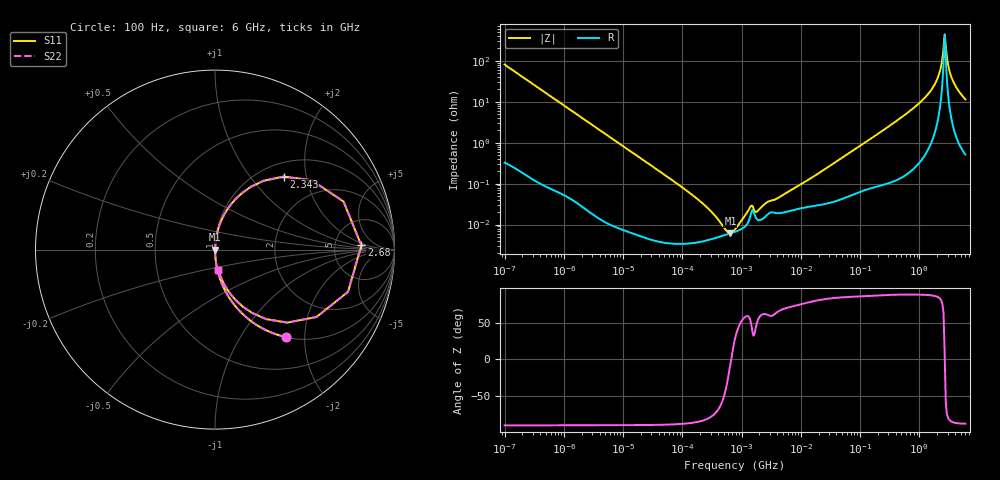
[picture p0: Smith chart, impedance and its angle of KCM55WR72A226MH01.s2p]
!Murata Part Number: KCM55WR72A226MH01
!These Parameters are Measured in Series Mode Connection
!Data Generated on Mar 13, 2026
!  o--ll--o
!Port1  Port2
!  o------o
!Operation Temp=25[degC], DC Bias Voltage=0[V]
!Freq. Start=100[Hz] Stop=6[GHz] 401[Steps]
# Hz S RI R 50
!Freq.(Hz) S11(Real) S11(Imag) S21(Real) S21(Imag) S12(Real) S12(Imag) S22(Real) S22(Imag)
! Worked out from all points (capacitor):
!   401 points, 100 Hz to 6 GHz, reference 50 ohm
!   read as one part in series: C = 19.6 uF near 109 Hz
!   lowest |Z| = 6.13 mohm at 647.6 kHz (marker M1)
!   series resonance near 665.1 kHz, so ESL is about 2.9 nH
!   S11 on the Smith chart (normalised r, x): 100 Hz: 1.01, -1.62; 2.343 GHz: 1.26, +1.49; 2.68 GHz: 9.67, +1.36; 6 GHz: 1.01, -0.23
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100  0.396 -0.4871  0.604 0.4871  0.604 0.4871  0.396 -0.4871
306  0.0666 -0.2471  0.9334 0.2471  0.9334 0.2471  0.0666 -0.2471
2008  0.00193 -0.0406  0.9981 0.0406  0.9981 0.0406  0.00193 -0.0406
40335  4.21e-05 -0.00204  1 0.00204  1 0.00204  4.21e-05 -0.00204
193316  3.74e-05 -0.000384  1 0.000384  1 0.000384  3.74e-05 -0.000384
452617  5.19e-05 -9.23e-05  0.9999 9.23e-05  0.9999 9.23e-05  5.19e-05 -9.23e-05
647581  6.1e-05 -6.1e-06  0.9999 6.1e-06  0.9999 6.1e-06  6.1e-05 -6.1e-06
774597  6.65e-05 3.55e-05  0.9999 -3.55e-05  0.9999 -3.55e-05  6.65e-05 3.55e-05
968953  7.6e-05 9.13e-05  0.9999 -9.13e-05  0.9999 -9.13e-05  7.6e-05 9.13e-05
1386327  0.00015 0.000214  0.9999 -0.000214  0.9999 -0.000214  0.00015 0.000214
1813585  0.000135 0.000158  0.9999 -0.000158  0.9999 -0.000158  0.000135 0.000158
1.555665e7  0.000281 0.00139  0.9997 -0.00139  0.9997 -0.00139  0.000281 0.00139
3.124326e8  0.00168 0.0255  0.9983 -0.0255  0.9983 -0.0255  0.00168 0.0255
9.150511e8  0.00947 0.0815  0.9905 -0.0815  0.9905 -0.0815  0.00947 0.0815
1.637704e9  0.0502 0.1932  0.9498 -0.1932  0.9498 -0.1932  0.0502 0.1932
2.048624e9  0.1495 0.3142  0.8505 -0.3142  0.8505 -0.3142  0.1495 0.3142
2.34314e9  0.382 0.4067  0.618 -0.4067  0.618 -0.4067  0.382 0.4067
2.679998e9  0.8156 0.0235  0.1844 -0.0235  0.1844 -0.0235  0.8156 0.0235
2.931063e9  0.5658 -0.3753  0.4342 0.3753  0.4342 0.3753  0.5658 -0.3753
3.205649e9  0.2852 -0.3874  0.7148 0.3874  0.7148 0.3874  0.2852 -0.3874
3.8344e9  0.0926 -0.2557  0.9074 0.2557  0.9074 0.2557  0.0926 -0.2557
6e9  0.0178 -0.1116  0.9822 0.1116  0.9822 0.1116  0.0178 -0.1116
